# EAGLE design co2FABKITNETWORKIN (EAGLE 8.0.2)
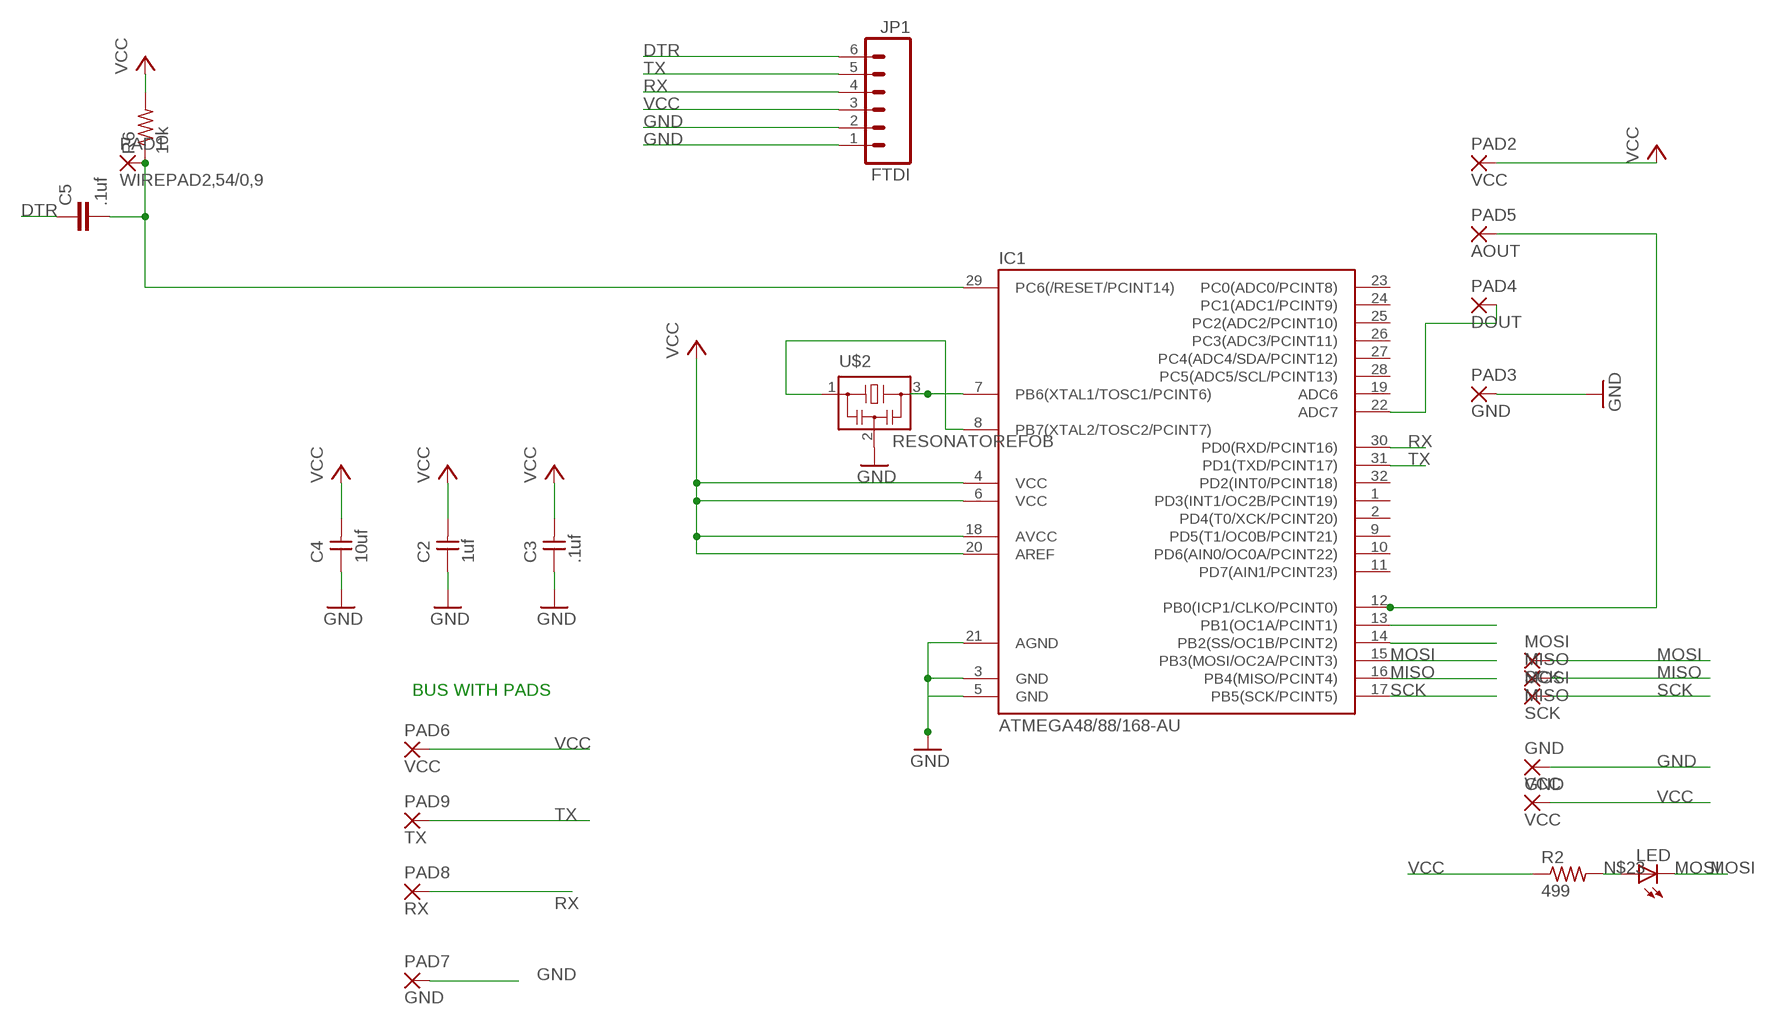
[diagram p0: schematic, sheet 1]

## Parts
C2  1uf  UNPOLARIZED_CAPACITOR1206  [1206]
C3  .1uf  UNPOLARIZED_CAPACITOR1206  [1206]
C4  10uf  UNPOLARIZED_CAPACITOR1206  [1206]
C5  .1uf  C-EUC1206  [C1206]
GND  GND  WIREPAD2,54/0,9  [2,54/0,9]
IC1  ATMEGA48/88/168-AU  [TQFP32-08]
JP1  FTDI  M06SMD  [1X06-SMD]
LED  LED1206  [1206]
MISO  MISO  WIREPAD2,54/0,9  [2,54/0,9]
MOSI  MOSI  WIREPAD2,54/0,9  [2,54/0,9]
PAD1  WIREPAD2,54/0,9  [2,54/0,9]
PAD2  VCC  WIREPAD2,54/0,9  [2,54/0,9]
PAD3  GND  WIREPAD2,54/0,9  [2,54/0,9]
PAD4  DOUT  WIREPAD2,54/0,9  [2,54/0,9]
PAD5  AOUT  WIREPAD2,54/0,9  [2,54/0,9]
PAD6  VCC  WIREPAD2,54/0,9  [2,54/0,9]
PAD7  GND  WIREPAD2,54/0,9  [2,54/0,9]
PAD8  RX  WIREPAD2,54/0,9  [2,54/0,9]
PAD9  TX  WIREPAD2,54/0,9  [2,54/0,9]
R2  499  RESISTOR1206  [1206]
R6  10k  RESISTOR1206  [1206]
SCK  SCK  WIREPAD2,54/0,9  [2,54/0,9]
U$2  RESONATOREFOB  [EFOBM]
VCC  VCC  WIREPAD2,54/0,9  [2,54/0,9]

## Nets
DTR: C5.1 JP1.6
GND: C2.1 C3.1 C4.1 GND.1(P) IC1.3(GND) IC1.5(GND) IC1.21(AGND) JP1.1 JP1.2 PAD3.1(P) PAD7.1(P) U$2.2
MISO: IC1.16(PB4(MISO/PCINT4)) MISO.1(P)
MOSI: IC1.15(PB3(MOSI/OC2A/PCINT3)) LED.2(C) MOSI.1(P)
N$1: IC1.8(PB7(XTAL2/TOSC2/PCINT7)) U$2.1
N$2: IC1.12(PB0(ICP1/CLKO/PCINT0)) PAD5.1(P)
N$3: IC1.22(ADC7) PAD4.1(P)
N$9: IC1.7(PB6(XTAL1/TOSC1/PCINT6)) U$2.3
N$17: IC1.13(PB1(OC1A/PCINT1))
N$18: IC1.14(PB2(SS/OC1B/PCINT2))
N$23: LED.1(A) R2.2
RST1: C5.2 IC1.29(PC6(/RESET/PCINT14)) PAD1.1(P) R6.1
RX: IC1.30(PD0(RXD/PCINT16)) JP1.4 PAD8.1(P)
SCK: IC1.17(PB5(SCK/PCINT5)) SCK.1(P)
TX: IC1.31(PD1(TXD/PCINT17)) JP1.5 PAD9.1(P)
VCC: C2.2 C3.2 C4.2 IC1.4(VCC) IC1.6(VCC) IC1.18(AVCC) IC1.20(AREF) JP1.3 PAD2.1(P) PAD6.1(P) R2.1 R6.2 VCC.1(P)
Unconnected: IC1.1(PD3(INT1/OC2B/PCINT19)) IC1.2(PD4(T0/XCK/PCINT20)) IC1.9(PD5(T1/OC0B/PCINT21)) IC1.10(PD6(AIN0/OC0A/PCINT22)) IC1.11(PD7(AIN1/PCINT23)) IC1.19(ADC6) IC1.23(PC0(ADC0/PCINT8)) IC1.24(PC1(ADC1/PCINT9)) IC1.25(PC2(ADC2/PCINT10)) IC1.26(PC3(ADC3/PCINT11)) IC1.27(PC4(ADC4/SDA/PCINT12)) IC1.28(PC5(ADC5/SCL/PCINT13)) IC1.32(PD2(INT0/PCINT18))

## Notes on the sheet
- BUS WITH PADS

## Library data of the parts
C2-C4 = ng:UNPOLARIZED_CAPACITOR: unpolarized_capacitor
C5 = rcl:C-EU: CAPACITOR, European symbol
GND MISO MOSI PAD1-PAD9 SCK VCC = wirepad:WIREPAD: Wire PAD connect wire on PCB
IC1 = atmega8:ATMEGA48/88/168
JP1 = SparkFun:M06: Header 6 Standard 6-pin 0.1" header. Use with straight break away headers (SKU : PRT-00116), right angle break away headers (PRT-00553), swiss pins (PRT-00743), machine pins (PRT-00117), and female headers (PRT-00115). Molex polarized connector foot print use with SKU : PRT-08094 with associated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
LED = ng:LED
R2 R6 = ng:RESISTOR
U$2 = fab:RESONATOR

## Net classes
0 Default: width 0.203 mm
1 VCC: width 0.254 mm

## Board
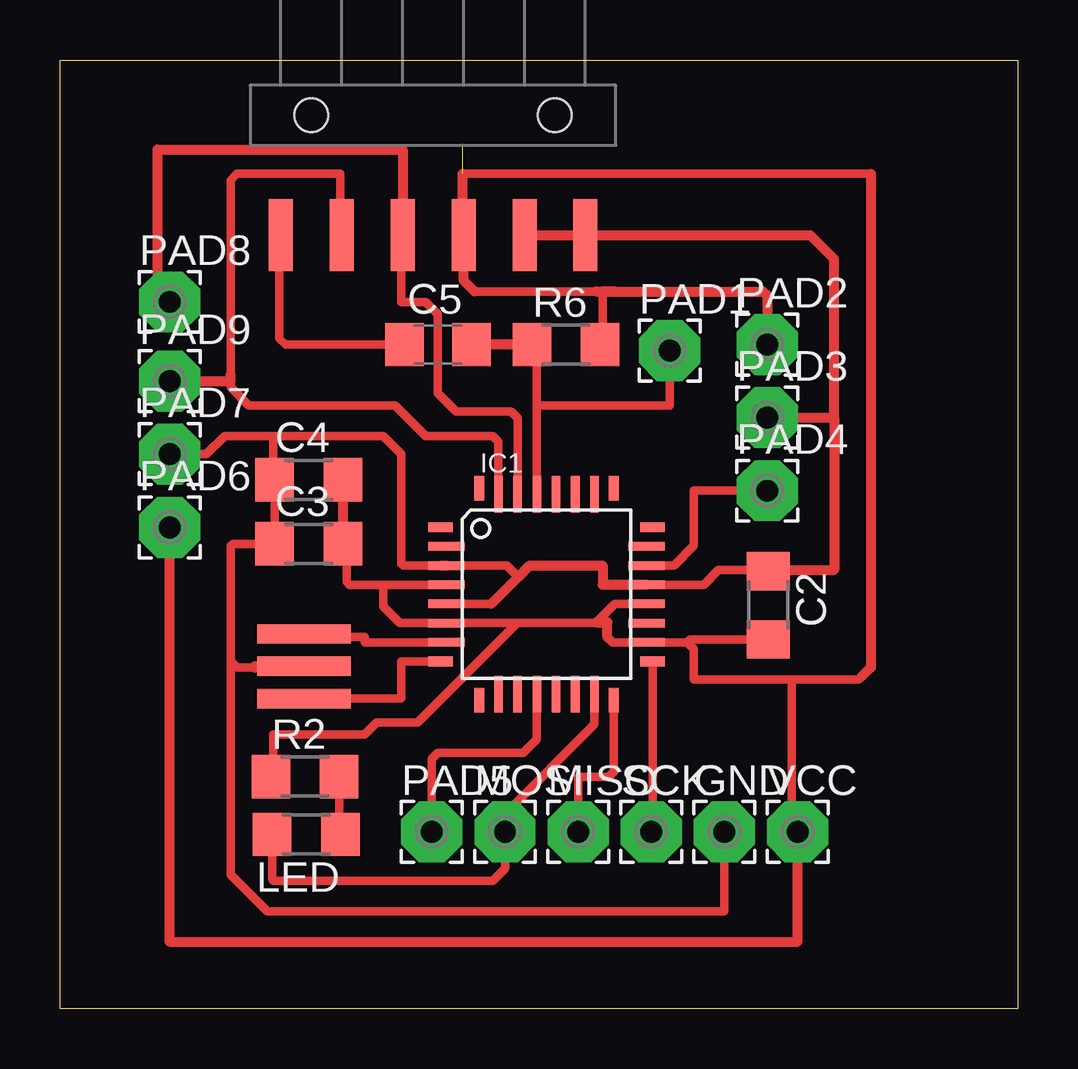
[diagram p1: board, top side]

Size 39.9 x 39.55 mm. Coordinates in mm from the lower left corner, seen from the top.
Outline: 0,39.55 39.9,39.55 39.9,0 0,0 0,39.55
Copper layers (1*16): Top 0.035mm / dielectric 1.5mm / Bottom 0.035mm
Design rules "default *": minimum track width 10mil, minimum drill 24mil, track to track 16mil, track to pad 16mil, pad to pad 16mil, via to via 16mil, smd to smd 16mil, copper to edge 16mil, drill to drill 8mil, minimum pad ring 10mil, minimum via ring 8mil, stop-mask expansion 4mil, vias tented up to drill 0mil, thermal gap 10mil

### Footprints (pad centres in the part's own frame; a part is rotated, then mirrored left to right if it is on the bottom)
1206 = smd 1.6 x 1.803: 1 -1.422,0; 2 1.422,0
C1206 = smd 1.6 x 1.8: 1 -1.4,0; 2 1.4,0
2,54/0,9 = drill 0.914 pad 2.54 octagon: 1 0,0
TQFP32-08 = smd 1.016 x 0.406: 1 -4.42,2.8; 8 -4.42,-2.8; 17 4.42,-2.8; 24 4.42,2.8 | smd 1.524 x 0.356: 2 -4.166,2; 3 -4.166,1.2; 4 -4.166,0.4; 5 -4.166,-0.4; 6 -4.166,-1.2; 7 -4.166,-2; 18 4.166,-2; 19 4.166,-1.2; 20 4.166,-0.4; 21 4.166,0.4; 22 4.166,1.2; 23 4.166,2 | smd 0.406 x 1.016: 9 -2.8,-4.42; 16 2.8,-4.42; 25 2.8,4.42; 32 -2.8,4.42 | smd 0.356 x 1.524: 10 -2,-4.166; 11 -1.2,-4.166; 12 -0.4,-4.166; 13 0.4,-4.166; 14 1.2,-4.166; 15 2,-4.166; 26 2,4.166; 27 1.2,4.166; 28 0.4,4.166; 29 -0.4,4.166; 30 -1.2,4.166; 31 -2,4.166
1X06-SMD = smd 1 x 3: 1 -6.35,5; 2 -3.81,5; 3 -1.27,5; 4 1.27,5; 5 3.81,5; 6 6.35,5 | hole 1.4: -5.08,0; 5.08,0
EFOBM = smd 0.8 x 3.9: 1 -1.35,0; 2 0,0; 3 1.35,0

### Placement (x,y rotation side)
C2  29.51,16.81 270 top
C3  10.36,19.38 0 top
C4  10.36,22.05 0 top
C5  15.75,27.69 0 top
GND  27.69,7.37 0 top
IC1  20.27,17.27 0 top
JP1  15.54,37.24 180 top
LED  10.26,7.26 180 top
MISO  21.59,7.37 0 top
MOSI  18.54,7.37 0 top
PAD1  25.4,27.43 0 top
PAD2  29.46,27.69 0 top
PAD3  29.46,24.64 0 top
PAD4  29.46,21.59 0 top
PAD5  15.49,7.37 0 top
PAD6  4.57,20.07 0 top
PAD7  4.57,23.11 0 top
PAD8  4.57,29.46 0 top
PAD9  4.57,26.16 0 top
R2  10.21,9.68 0 top
R6  21.08,27.69 0 top
SCK  24.64,7.37 0 top
U$2  10.16,14.27 90 top
VCC  30.73,7.37 0 top

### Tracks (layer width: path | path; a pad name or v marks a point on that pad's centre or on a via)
DTR
  Top 0.356: C5.1 9.4,27.69 9.14,27.94 9.14,32.19 JP1.6
GND
  Top 0.356: 24.33,17.68 24.33,17.67 IC1.21 26.82,17.67 27.43,18.29 29.46,18.29 C2.1 | IC1.5 17.96,16.87 | 19.09,18 18.61,18.47 IC1.3 14.29,18.47 14.22,18.54 14.22,23.11 13.46,23.88 8.89,23.88 | 8.89,23.88 8.89,22.1 C4.1 C3.1 7.19,19.38 7.11,19.3 7.11,14.48 | PAD7.1 6.1,23.11 6.86,23.88 8.89,23.88 | 7.11,14.48 7.37,14.22 8.13,14.22 10.11,14.22 U$2.2 | GND.1 27.69,4.06 8.64,4.06 7.11,5.59 7.11,14.48
  Top 0.406: 15.9,18.47 15.93,18.47 | 15.93,18.47 IC1.3 | 15.93,18.47 | IC1.21 22.61,17.68 22.61,18.47 19.56,18.47 19.09,18 17.96,16.87 | JP1.2 JP1.1 31.26,32.24 32.26,31.24 32.26,24.64 | 32.26,24.64 32.26,18.29 29.57,18.29 C2.1 | PAD3.1 32.26,24.64 | U$2.2 8.13,14.28 8.13,14.22
MISO
  Top 0.305: IC1.16 23.07,12.49
  Top 0.356: IC1.16 23.07,9.86 22.86,9.65 21.59,9.65 21.59,7.62 | 21.59,7.62 MISO.1 21.59,7.62
  Top 0.406: 23.09,12.83 IC1.16
MOSI
  Top 0.356: IC1.15 22.27,11.86 18.54,8.13 MOSI.1 18.54,5.84 18.03,5.33 8.89,5.33 8.84,5.38 LED.2
N$1
  Top 0.356: U$2.1 14.22,12.93 14.22,14.48 14.22,14.47 IC1.8
N$2
  Top 0.356: IC1.12 19.87,11.23 19.3,10.67 15.75,10.67 15.49,10.41 PAD5.1
N$3
  Top 0.356: IC1.22 25.58,18.47 26.42,19.3 26.42,21.59 28.7,21.59 | 28.7,21.59 PAD4.1 28.7,21.59
N$9
  Top 0.356: 10.92,15.49 12.7,15.49 12.7,15.27 IC1.7 | 10.92,15.49 10.16,15.49 9.4,15.49 9.4,15.75 10.92,15.75 10.92,15.49
  Top 0.406: U$2.3 10.16,15.49
N$23
  Top 0.356: R2.2 11.63,8.08 LED.1
  Top 0.406: LED.1 11.94,7.95
RST1
  Top 0.356: C5.2 17.4,27.69 | 19.87,24.89 IC1.29 | 19.87,25.15 19.87,24.89 | 19.87,25.15 19.87,25.65 | 19.87,25.65 19.87,27.48 R6.1 | 19.87,25.65 19.87,25.15 | 19.87,25.15 19.87,24.89 | PAD1.1 25.4,25.15 19.87,25.15
  Top 0.406: R6.1 C5.2
RX
  Top 0.356: IC1.30 19.07,24.62 18.8,24.89 16.51,24.89 15.75,25.65 15.75,28.96 15.24,29.46 14.22,29.46 14.22,32.19 JP1.4
  Top 0.406: PAD8.1 4.06,29.46 4.06,35.81 14.28,35.81 JP1.4
SCK
  Top 0.356: SCK.1 24.69,7.42 IC1.17
TX
  Top 0.356: IC1.31 18.27,23.64 18.03,23.88 15.24,23.88 13.97,25.15 7.87,25.15 7.11,25.91 7.11,26.42 7.11,34.54 7.37,34.8 11.68,34.8 11.68,32.29 JP1.5
  Top 0.406: PAD9.1 7.11,26.16 7.11,26.42
VCC  (1 unrouted)
  Top 0.305: IC1.20
  Top 0.356: IC1.20 23.12,16.87 22.35,16.1 22.32,16.07 19.05,16.07 | IC1.18 | 22.61,29.9 22.61,27.84 R6.2 | 23.11,29.9 22.35,29.9 17.27,29.9 | 33.78,34.8 16.76,34.8 | 26.13,15.27 IC1.18 | 19.05,16.07 IC1.6 14.15,16.07 13.46,16.76 13.46,17.67 | 13.46,17.67 IC1.4 | 13.46,17.67 12.05,17.67 11.94,17.78 11.94,19.23 | IC1.18 23.03,15.27 22.81,15.49 | C2.2 26.25,15.39 26.13,15.27 | 26.13,15.27 26.42,14.99 26.42,13.72 30.48,13.72 | 30.48,13.72 33.27,13.72 33.4,13.84 | 30.48,13.72 30.48,7.62 VCC.1 | 19.05,16.07 14.92,11.94 13.21,11.94 12.7,11.43 8.89,11.43 8.89,9.78 R2.1
  Top 0.406: 22.35,16.1 22.81,16.1 22.81,15.49 | 23.11,29.9 22.61,29.9 | C4.2 C3.2 11.94,19.23 | 22.35,29.9 29.29,29.9 29.46,29.72 PAD2.1 | 33.78,34.8 33.78,14.22 33.4,13.84 | JP1.3 16.82,30.35 17.27,29.9 | JP1.3 16.76,32.29 16.76,33.02 | 16.76,34.8 16.76,33.02 | JP1.3 16.82,32.97 16.76,33.02 | VCC.1 30.73,2.79 4.57,2.79 PAD6.1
